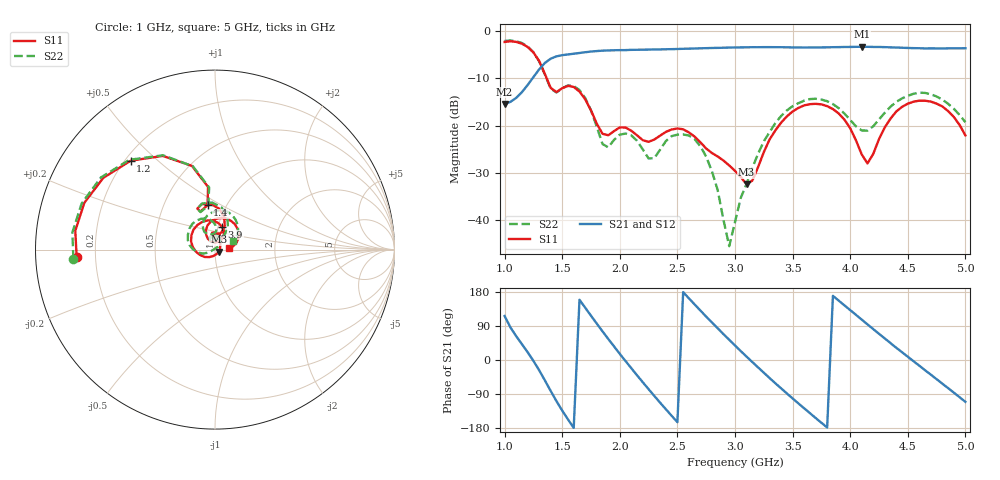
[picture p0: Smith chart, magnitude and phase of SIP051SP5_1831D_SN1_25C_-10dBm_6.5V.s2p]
# GHz  S  dB  R  50
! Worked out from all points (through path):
!   81 points, 1 GHz to 5 GHz, reference 50 ohm
!   highest |S21| = -3.27 dB at 4.1 GHz (marker M1); lowest = -15.4 dB at 1 GHz (marker M2)
!   lowest |S11| = -32.5 dB at 3.1 GHz (marker M3), VSWR 1.05, Z = 52.1 - j1.18 ohm
!   |S11| at or under -10 dB: 1.366 GHz to end of sweep
!   |S22| runs from -45.6 to -1.9 dB; largest |S21 - S12| = 0.0034
!   S11 on the Smith chart (normalised r, x): 1 GHz: 0.13, -0.03; 1.2 GHz: 0.22, +0.41; 1.4 GHz: 0.82, +0.43; 3.9 GHz: 1.04, +0.27; 5 GHz: 1.17, +0.02
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1  -2.25 -176.9  -15.45 116.0  -15.44 115.8  -2.04 -176.3
1.2  -3.31 133.5  -11.40 20.4  -11.39 20.6  -3.21 133.6
1.3  -6.31 105.4  -8.07 -27.1  -8.06 -27.1  -6.36 104.9
1.4  -12.01 99.5  -5.81 -81.7  -5.80 -81.7  -12.16 98.8
1.55  -11.58 106.3  -4.90 -156.8  -4.89 -156.8  -11.48 105.5
1.7  -14.44 74.4  -4.44 137.9  -4.45 138.0  -14.18 69.4
1.85  -21.76 80.4  -4.10 75.6  -4.10 75.6  -23.93 69.8
2.05  -20.43 94.4  -3.98 -2.9  -3.99 -2.9  -21.70 93.2
2.2  -23.12 91.7  -3.90 -58.9  -3.89 -58.8  -25.10 82.6
2.35  -22.15 104.2  -3.83 -112.7  -3.82 -112.6  -25.13 118.6
2.6  -21.46 71.3  -3.68 162.6  -3.68 162.7  -22.11 77.9
2.8  -25.85 55.5  -3.53 98.9  -3.53 98.9  -29.74 45.6
2.95  -28.48 40.4  -3.45 53.2  -3.44 53.3  -45.63 136.7
3  -29.63 28.5  -3.42 38.4  -3.42 38.3  -40.49 -172.8
3.1  -32.48 -28.4  -3.39 9.0  -3.38 9.0  -32.42 -159.1
3.4  -19.41 -173.7  -3.37 -74.7  -3.37 -74.8  -17.98 177.7
3.7  -15.40 114.3  -3.42 -153.0  -3.42 -152.9  -14.32 123.7
3.9  -17.44 73.4  -3.35 156.7  -3.35 156.7  -16.31 93.3
4.1  -26.14 64.0  -3.27 106.6  -3.27 106.6  -21.04 95.4
4.35  -18.54 115.3  -3.40 44.6  -3.40 44.7  -16.00 115.6
4.65  -14.74 60.9  -3.62 -27.0  -3.60 -26.8  -13.07 71.6
5  -22.09 6.3  -3.59 -110.4  -3.59 -110.3  -19.29 25.6
